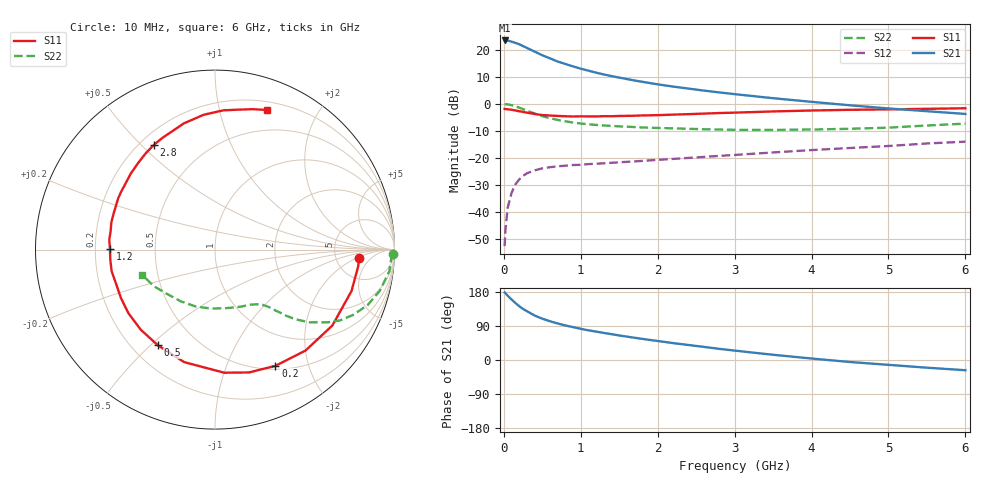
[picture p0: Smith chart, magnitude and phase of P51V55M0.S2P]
! SIEMENS Small Signal Semiconductors
! BFP183
! Si NPN RF Bipolar Junction Transistor in SOT143
! VCE = 1.5 V  IC = 5 mA
! Common Emitter S-Parameters:  March  1996
# GHz  S  MA  R  50
!  f  S11  S21  S12  S22
! GHz  MAG  ANG  MAG  ANG  MAG  ANG  MAG  ANG
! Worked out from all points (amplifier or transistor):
!   36 points, 10 MHz to 6 GHz, reference 50 ohm
!   highest |S21| = 23.5 dB at 10 MHz (marker M1)
!   |S21| within 3 dB of that: start of sweep to 317 MHz
!   unconditionally stable (mu >= 1): 1.518 GHz to 5.855 GHz
!   at 250 MHz: K = 0.21, MSG = 24.1 dB, |S12| = -26.7 dB
!   at 1.4 GHz: K = 0.96, MSG = 16.1 dB, |S12| = -21.8 dB
!   at 6 GHz: K = 0.98, MSG = 5.1 dB, |S12| = -14.0 dB
!   S11 on the Smith chart (normalised r, x): 10 MHz: 8.69, -2.30; 200 MHz: 0.54, -1.51; 500 MHz: 0.30, -0.53; 1.2 GHz: 0.26, +0.00; 2.8 GHz: 0.25, +0.55; 6 GHz: 0.28, +1.40
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0.01  0.8059 -3.3  15.01 178.2  0.0023 81.9  0.9929 -1.4
0.02  0.803 -6.8  14.92 176.4  0.0045 85.6  0.9835 -2.8
0.05  0.7949 -16.9  14.9 169.6  0.0119 82.4  0.9788 -7.1
0.1  0.7787 -32.9  14.29 159.8  0.0223 72.6  0.9469 -14.0
0.15  0.7555 -48.1  13.51 150.5  0.0322 65.6  0.9047 -20.0
0.2  0.7299 -62.5  12.79 142.0  0.0397 60.0  0.8526 -25.2
0.25  0.7103 -74.5  11.78 134.7  0.0462 54.5  0.8006 -29.5
0.3  0.6879 -85.7  10.91 128.8  0.0516 49.5  0.7496 -32.7
0.4  0.65 -105.3  9.325 117.4  0.0586 43.3  0.6622 -37.7
0.5  0.621 -120.8  7.974 109.0  0.0638 38.0  0.593 -40.9
0.6  0.6085 -132.9  6.982 102.2  0.067 35.1  0.5419 -42.9
0.7  0.5984 -143.7  6.106 96.4  0.0696 32.9  0.5048 -44.1
0.9  0.5832 -160.9  4.958 86.7  0.0735 30.4  0.4514 -46.2
1.1  0.5861 -174.5  4.131 78.3  0.0765 29.1  0.4182 -48.3
1.2  0.5852 179.8  3.794 74.9  0.0777 28.5  0.4075 -49.2
1.7  0.6036 156.1  2.714 58.7  0.0858 29.2  0.3715 -55.6
2.2  0.6322 137.9  2.096 44.6  0.0954 30.0  0.3519 -63.9
2.8  0.6763 120.1  1.633 29.4  0.1085 30.1  0.3342 -76.5
3.5  0.7245 103.8  1.275 13.8  0.1258 29.1  0.3291 -94.0
4.5  0.7772 86.6  0.942 -5.3  0.1522 24.9  0.3454 -123.4
5.5  0.8102 74.9  0.732 -20.3  0.1845 19.8  0.3974 -149.2
6  0.8302 69.6  0.651 -27.0  0.1993 15.8  0.4305 -161.1
